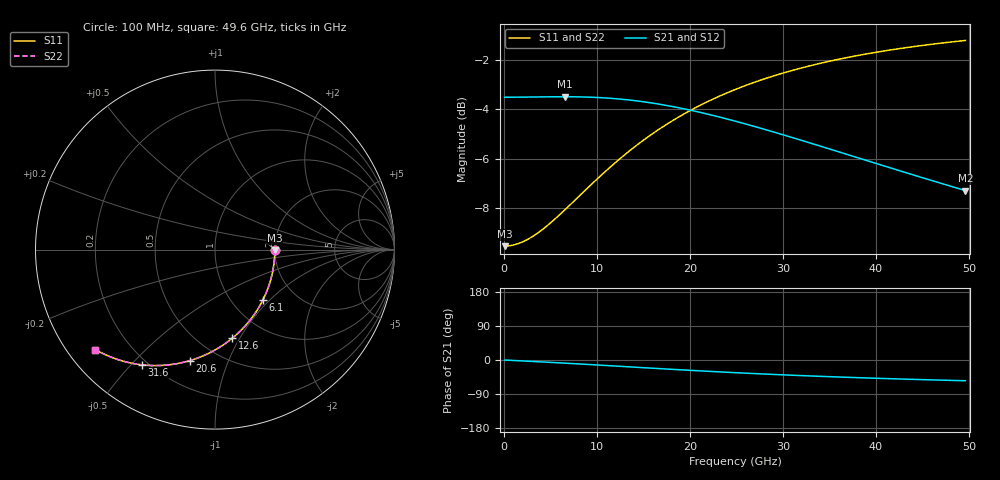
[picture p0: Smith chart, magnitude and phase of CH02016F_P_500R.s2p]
# GHz S RI R 500
! S-Parameters data
! Freq  reS11  imS11  reS21  imS21  reS12  imS12  reS22  imS22
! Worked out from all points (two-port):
!   100 points, 100 MHz to 49.6 GHz, reference 500 ohm
!   highest |S21| = -3.50 dB at 6.6 GHz (marker M1); lowest = -7.3 dB at 49.6 GHz (marker M2)
!   |S21| within 3 dB of the highest: start of sweep to 42.62 GHz
!   lowest |S11| = -9.5 dB at 100 MHz (marker M3), VSWR 2.00, Z = 1e+03 - j11 ohm
!   |S11| at or under -10 dB: nowhere
!   |S22| runs from -9.5 to -1.2 dB; largest |S21 - S12| = 0
!   S11 on the Smith chart (normalised r, x): 100 MHz: 2.00, -0.02; 6.1 GHz: 1.38, -0.91; 12.6 GHz: 0.71, -0.93; 20.6 GHz: 0.35, -0.73; 31.6 GHz: 0.18, -0.54; 49.6 GHz: 0.08, -0.36
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0.1  0.3333 -0.00487  0.6667 -0.00141  0.6667 -0.00141  0.3333 -0.00487
1.6  0.3285 -0.0776  0.6665 -0.0227  0.6665 -0.0227  0.3285 -0.0776
3.1  0.3154 -0.1487  0.6658 -0.0443  0.6658 -0.0443  0.3154 -0.1487
4.6  0.2946 -0.2167  0.6645 -0.0664  0.6645 -0.0664  0.2946 -0.2167
6.1  0.267 -0.2805  0.6621 -0.0892  0.6621 -0.0892  0.267 -0.2805
6.6  0.2565 -0.3006  0.661 -0.097  0.661 -0.097  0.2565 -0.3006
8.6  0.2091 -0.3752  0.6549 -0.1284  0.6549 -0.1284  0.2091 -0.3752
10.6  0.1549 -0.4395  0.6454 -0.1601  0.6454 -0.1601  0.1549 -0.4395
12.6  0.0967 -0.4934  0.6324 -0.1911  0.6324 -0.1911  0.0967 -0.4934
14.6  0.0364 -0.5374  0.616 -0.2205  0.616 -0.2205  0.0364 -0.5374
16.6  -0.0242 -0.5723  0.5965 -0.2477  0.5965 -0.2477  -0.0242 -0.5723
18.6  -0.0838 -0.5991  0.5747 -0.2721  0.5747 -0.2721  -0.0838 -0.5991
20.6  -0.1415 -0.6188  0.5511 -0.2934  0.5511 -0.2934  -0.1415 -0.6188
22.6  -0.1967 -0.6325  0.5264 -0.3116  0.5264 -0.3116  -0.1967 -0.6325
25.1  -0.2617 -0.6425  0.4949 -0.33  0.4949 -0.33  -0.2617 -0.6425
28.1  -0.3332 -0.6461  0.4573 -0.3461  0.4573 -0.3461  -0.3332 -0.6461
31.6  -0.4078 -0.6418  0.4151 -0.3581  0.4151 -0.3581  -0.4078 -0.6418
33.1  -0.437 -0.6379  0.3979 -0.3613  0.3979 -0.3613  -0.437 -0.6379
37.1  -0.5069 -0.623  0.3549 -0.3654  0.3549 -0.3654  -0.5069 -0.623
41.6  -0.5735 -0.6012  0.3121 -0.364  0.3121 -0.364  -0.5735 -0.6012
45.6  -0.6235 -0.5794  0.2787 -0.3593  0.2787 -0.3593  -0.6235 -0.5794
49.6  -0.6661 -0.5567  0.2495 -0.3523  0.2495 -0.3523  -0.6661 -0.5567
